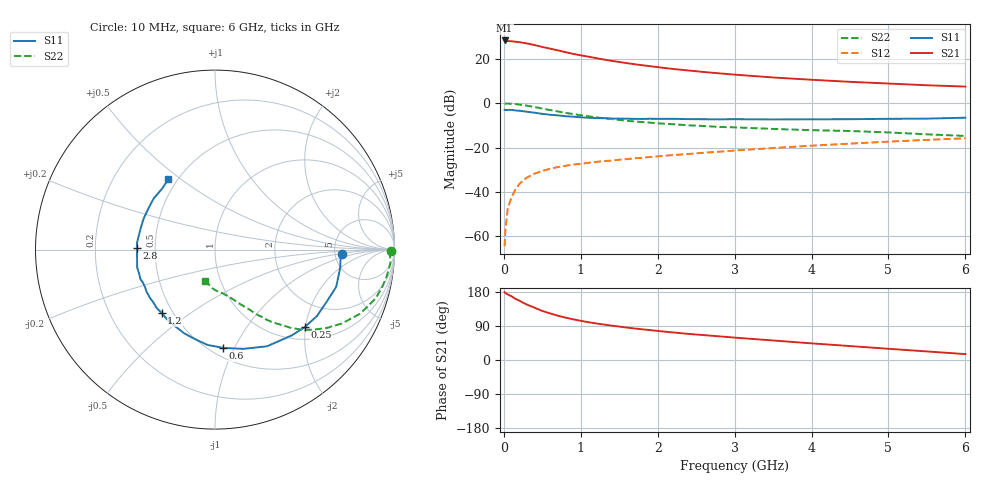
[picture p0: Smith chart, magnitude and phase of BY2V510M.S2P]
! SIEMENS Small Signal Semiconductors
! BFY420
! Si NPN RF SIEGET Grounded Emitter Transistor in MICRO-X
! VCE = 2.5 V  IC = 10 mA
! Common Emitter S-Parameters:  October  1996
# GHz  S  MA  R  50
!  f  S11  S21  S12  S22
! GHz  MAG  ANG  MAG  ANG  MAG  ANG  MAG  ANG
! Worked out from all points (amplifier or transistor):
!   36 points, 10 MHz to 6 GHz, reference 50 ohm
!   highest |S21| = 28.3 dB at 10 MHz (marker M1)
!   |S21| within 3 dB of that: start of sweep to 508.5 MHz
!   unconditionally stable (mu >= 1): 2.529 GHz to end of sweep
!   at 250 MHz: K = 0.19, MSG = 31.0 dB, |S12| = -34.8 dB
!   at 1.4 GHz: K = 0.75, MSG = 22.5 dB, |S12| = -25.9 dB
!   at 6 GHz: K = 1.09, MAG = 9.8 dB, |S12| = -15.8 dB
!   S11 on the Smith chart (normalised r, x): 10 MHz: 5.79, -0.51; 250 MHz: 1.29, -1.98; 600 MHz: 0.58, -0.91; 1.2 GHz: 0.44, -0.39; 2.8 GHz: 0.39, +0.01; 6 GHz: 0.45, +0.45
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0.01  0.7073 -1.8  25.96 179.2  0.0006 103.7  0.9802 -0.6
0.02  0.7012 -3.6  25.75 176.7  0.0014 85.9  0.9744 -1.5
0.05  0.7051 -8.2  25.19 173.1  0.0042 88.3  0.9804 -4.2
0.1  0.7064 -17.1  24.92 168.1  0.0076 82.1  0.9692 -8.7
0.15  0.6863 -25.3  24.34 161.5  0.0113 77.1  0.9536 -12.9
0.2  0.6778 -33.1  23.77 156.8  0.015 75.0  0.9355 -16.8
0.25  0.6607 -40.9  23.05 151.1  0.0181 70.6  0.9067 -20.6
0.3  0.6414 -48.2  22.23 146.2  0.0211 68.7  0.8809 -24.1
0.4  0.6118 -61.7  20.45 138.0  0.0258 63.6  0.8183 -30.2
0.5  0.5752 -74.0  18.51 129.4  0.0298 59.2  0.7586 -35.2
0.6  0.5496 -85.2  17.02 123.0  0.0332 56.6  0.7023 -39.5
0.8  0.5097 -103.1  14.17 111.9  0.0388 51.7  0.6072 -45.9
0.9  0.4971 -110.2  12.96 107.4  0.0415 50.8  0.5691 -48.0
1.1  0.4714 -124.6  11.19 99.8  0.0454 49.9  0.5072 -52.2
1.2  0.4612 -130.1  10.38 96.4  0.0476 49.6  0.4806 -53.9
1.6  0.4478 -148.4  7.984 85.4  0.055 48.4  0.4018 -59.0
2.2  0.445 -166.9  5.912 72.7  0.0679 47.3  0.336 -65.1
2.8  0.4338 178.9  4.713 62.4  0.0807 45.9  0.2923 -70.3
3.5  0.4308 165.0  3.803 51.5  0.0975 43.1  0.2633 -76.0
4.5  0.4363 148.1  3.034 36.8  0.1229 36.9  0.2365 -85.2
5.5  0.4497 130.9  2.539 22.6  0.1493 29.2  0.1992 -99.2
6  0.471 123.4  2.372 15.6  0.162 24.7  0.1827 -108.4
